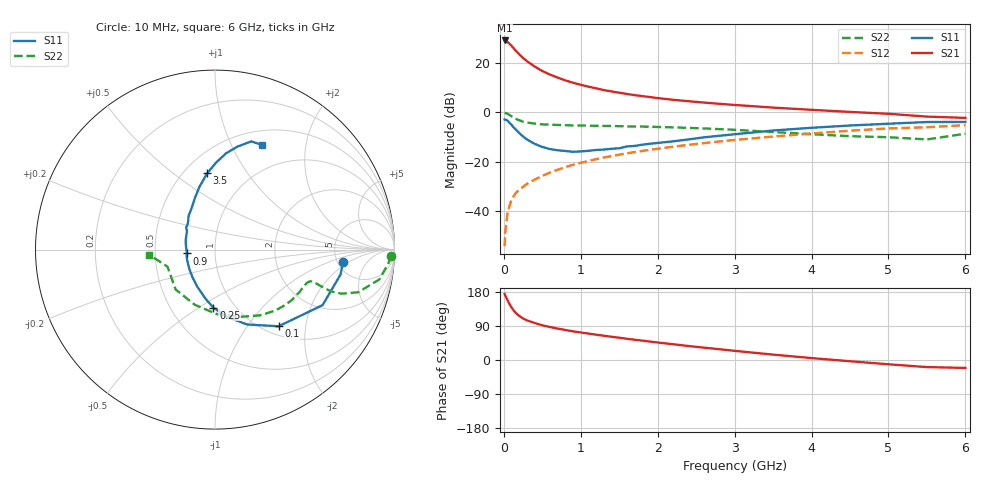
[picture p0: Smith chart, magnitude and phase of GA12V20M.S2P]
! Infineon Technologies  Discrete & RF Semiconductors
! BF775
! Si NPN RF Bipolar Junction Transistor in SOT23
! VCE = 12 V  IC = 20 mA
! Common Emitter S-Parameters:  May  1996
# GHz  S  MA  R  50
!  f  S11  S21  S12  S22
! GHz  MAG  ANG  MAG  ANG  MAG  ANG  MAG  ANG
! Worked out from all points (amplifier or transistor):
!   36 points, 10 MHz to 6 GHz, reference 50 ohm
!   highest |S21| = 29.2 dB at 10 MHz (marker M1)
!   |S21| within 3 dB of that: start of sweep to 123 MHz
!   unconditionally stable (mu >= 1): 465.9 MHz to 2.553 GHz
!   at 250 MHz: K = 0.80, MSG = 26.2 dB, |S12| = -30.3 dB
!   at 1.4 GHz: K = 1.09, MAG = 11.3 dB, |S12| = -17.8 dB
!   at 6 GHz: K = 0.87, MSG = 1.5 dB, |S12| = -5.2 dB
!   S11 on the Smith chart (normalised r, x): 10 MHz: 5.60, -1.62; 100 MHz: 1.16, -1.43; 250 MHz: 0.80, -0.58; 900 MHz: 0.73, -0.03; 3.5 GHz: 0.64, +0.67; 6 GHz: 0.67, +1.31
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0.01  0.7175 -5.6  28.99 174.2  0.0019 87.4  0.9807 -2.0
0.02  0.7128 -11.3  28.5 169.5  0.0039 84.0  0.9701 -4.4
0.05  0.6746 -27.3  26.85 156.5  0.0095 76.7  0.9307 -10.3
0.1  0.5551 -50.3  22.59 138.3  0.0169 69.4  0.832 -16.6
0.15  0.4545 -66.7  18.33 125.1  0.0224 65.9  0.7469 -19.2
0.2  0.3795 -80.3  15.22 116.3  0.0269 65.1  0.6886 -19.8
0.25  0.3233 -91.6  12.8 109.5  0.0306 66.0  0.6472 -19.4
0.3  0.2819 -100.2  11 104.6  0.0351 66.9  0.6218 -19.0
0.4  0.2292 -115.5  8.557 97.7  0.0429 67.9  0.5902 -18.4
0.5  0.1976 -129.8  6.929 91.5  0.0511 68.9  0.5707 -18.2
0.6  0.1792 -142.8  5.866 87.0  0.0597 70.0  0.56 -18.3
0.7  0.1695 -153.1  5.089 82.9  0.0681 70.4  0.5543 -18.8
0.8  0.1638 -164.5  4.465 79.2  0.0772 70.0  0.5476 -19.5
0.9  0.158 -172.2  3.999 75.7  0.0859 69.9  0.5424 -20.4
1.1  0.1652 169.6  3.332 69.8  0.1027 69.3  0.5359 -22.7
1.3  0.1752 156.9  2.841 64.1  0.1207 68.3  0.5297 -25.0
1.6  0.2025 142.5  2.362 56.0  0.1468 66.0  0.5194 -29.3
2.2  0.2572 121.6  1.801 41.6  0.2004 61.3  0.4946 -39.3
3.5  0.4272 95.9  1.249 14.2  0.3221 48.2  0.3985 -70.1
4.5  0.5404 83.4  1.021 -3.3  0.4238 36.1  0.3275 -110.1
5.5  0.6359 71.5  0.82 -18.7  0.4987 20.2  0.2815 -160.4
6  0.6394 66.0  0.772 -20.9  0.5499 15.8  0.3676 -175.5
